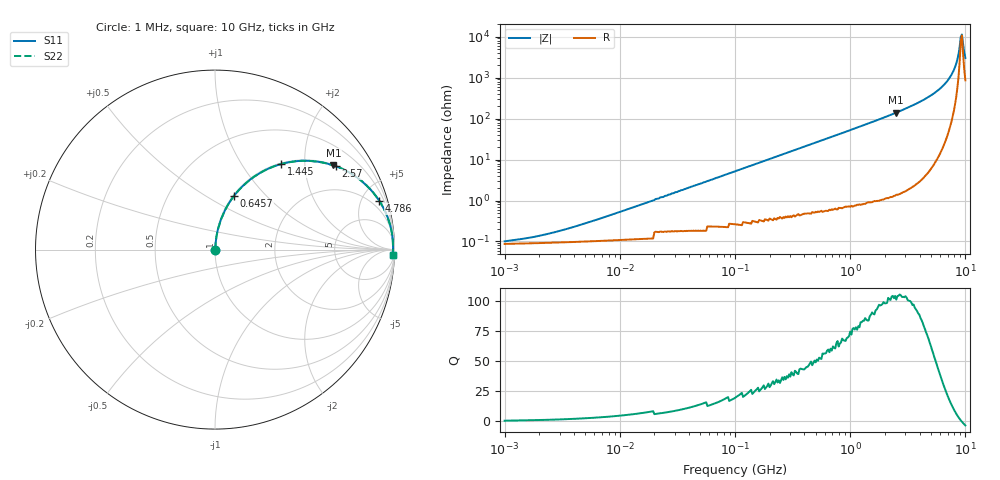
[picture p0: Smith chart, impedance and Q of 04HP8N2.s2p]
# MHz S MA R 50
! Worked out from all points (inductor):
!   401 points, 1 MHz to 10 GHz, reference 50 ohm
!   read as one part in series: L = 8.2 nH near 6.026 MHz
!   highest Q = 104 at 2.512 GHz (marker M1), where L = 8.85 nH
!   self-resonance near 9.12 GHz
!   S11 on the Smith chart (normalised r, x): 1 MHz: 1.00, +0.00; 645.7 MHz: 1.01, +0.67; 1.445 GHz: 1.02, +1.53; 2.57 GHz: 1.03, +2.87; 4.786 GHz: 1.09, +6.73; 10 GHz: 18, -58
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1  0.0009043 34.7  0.999 -0.0  0.999 -0.0  0.0009043 34.7
2.042  0.00134 51.6  0.999 -0.1  0.999 -0.1  0.00134 51.6
4.677  0.002599 67.7  0.999 -0.1  0.999 -0.1  0.002599 67.7
21.878  0.011 81.8  0.998 -0.6  0.998 -0.6  0.011 81.8
102.329  0.053 84.2  0.996 -3.0  0.996 -3.0  0.053 84.2
467.735  0.234 75.3  0.967 -13.5  0.967 -13.5  0.234 75.3
645.654  0.315 70.6  0.944 -18.4  0.944 -18.4  0.315 70.6
977.237  0.451 62.4  0.886 -26.8  0.886 -26.8  0.451 62.4
1445.44  0.603 52.2  0.79 -37.1  0.79 -37.1  0.603 52.2
2187.762  0.763 39.7  0.639 -49.7  0.639 -49.7  0.763 39.7
2511.886  0.809 35.4  0.579 -54.0  0.579 -54.0  0.809 35.4
2570.396  0.817 34.7  0.569 -54.8  0.569 -54.8  0.817 34.7
4786.301  0.955 16.5  0.284 -72.7  0.284 -72.7  0.955 16.5
6165.95  0.98 9.9  0.172 -78.5  0.172 -78.5  0.98 9.9
7413.102  0.99 5.4  0.093 -81.0  0.093 -81.0  0.99 5.4
7943.282  0.991 3.7  0.065 -80.5  0.065 -80.5  0.991 3.7
8317.638  0.992 2.6  0.046 -78.6  0.046 -78.6  0.992 2.6
8912.509  0.992 0.9  0.018 -63.6  0.018 -63.6  0.992 0.9
9120.108  0.992 0.4  0.01 -39.5  0.01 -39.5  0.992 0.4
9332.543  0.992 -0.2  0.008815 18.6  0.008815 18.6  0.992 -0.2
9549.926  0.991 -0.7  0.015 54.3  0.015 54.3  0.991 -0.7
10000  0.99 -1.8  0.033 71.6  0.033 71.6  0.99 -1.8
